TYPE ConfigPurge :
STRUCT
	PurgeCycleCount:SVINT;
	
	PurgeVentPressure:SVINT;
	PurgePumpPressure:SVINT;
	
	PurgeVentTimeLimit:SVINT;
	PurgePumpTimeLimit:SVINT;
	
	PurgeVentStableTime:SVINT;
	PurgePumpTime:SVINT;
	
	GasPurgeCycleCount:SVINT;
	GasPurgeFlowTime:SVINT;
	GasPurgePumpTime:SVINT;
END_STRUCT
END_TYPE
